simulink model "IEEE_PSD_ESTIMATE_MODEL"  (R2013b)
settings: Solver=ode45  StartTime=0.0  StopTime=SimulationDuration  RelTol=1e-3
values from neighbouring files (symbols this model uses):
  Amplitude = TypicalTransmitAmplitude * 0.95    (= 1.14)    [IEEE_PSD_ESTIMATE.m]
  Coefficients = [1 1 1 1 1 1] / 6    [IEEE_PSD_ESTIMATE.m]
  CouplingFilterFrequency = 8e6    (= 8000000)    [IEEE_PSD_ESTIMATE.m]
  DataRate = 10e6    (= 10000000)    [IEEE_PSD_ESTIMATE.m]
  Oversampling = 8    [IEEE_PSD_ESTIMATE.m]
  SymbolRate = DataRate * 3 / 4    (= 7500000)    [IEEE_PSD_ESTIMATE.m]
  Termination = 100    [IEEE_PSD_ESTIMATE.m]
  TransmitFilterFrequency = 12e6    (= 12000000)    [IEEE_PSD_ESTIMATE.m]
libraries: dspsigops x1, commrandsrc2 x1

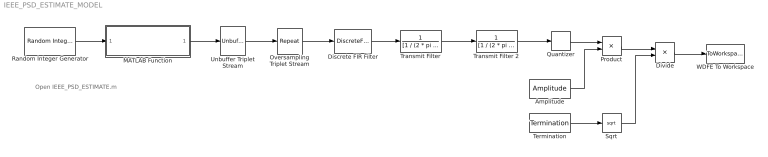
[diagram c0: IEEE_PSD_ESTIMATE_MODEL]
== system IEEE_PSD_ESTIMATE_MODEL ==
  note: Open IEEE_PSD_ESTIMATE.m
  Amplitude : Constant  Value=Amplitude
  Discrete FIR Filter : DiscreteFir  Coefficients=Coefficients
  Divide : Product  Inputs=*/
  MATLAB Function : MATLAB Function  TreatAsAtomicUnit=on
  Oversampling Triplet Stream : dspsigops/Repeat  N=16  RateOptions=Allow multirate processing  ic=0  mode=Unused parameter value
  Product : Product
  Quantizer : Quantizer  QuantizationInterval=1e-9  SampleTime=1 / (Oversampling * SymbolRate)
  Random Integer Generator : commrandsrc2/Random Integer Generator  mul=16  seed=37  Ts=4 / DataRate  frameBased=off  sampPerFrame=1  orient=off  outDataType=double
  Sqrt : Sqrt
  Termination : Constant  Value=Termination
  Transmit Filter : TransferFcn  Numerator=1  Denominator=[1 / (2 * pi * TransmitFilterFrequency) 1]
  Transmit Filter 2 : TransferFcn  Numerator=1  Denominator=[1 / (2 * pi * CouplingFilterFrequency) 1]
  Unbuffer Triplet Stream : Unbuffer  SampleBasedProcessing=Same as frame based
  WDFE To Workspace : ToWorkspace  VariableName=TX  SampleTime=-1
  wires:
  MATLAB Function/1(Triplet) -> Unbuffer Triplet Stream/1
  Unbuffer Triplet Stream/1 -> Oversampling Triplet Stream/1
  Random Integer Generator/1 -> MATLAB Function/1(Nibble)
  Oversampling Triplet Stream/1 -> Discrete FIR Filter/1
  Discrete FIR Filter/1 -> Transmit Filter/1
  Product/1 -> Divide/1
  Divide/1 -> WDFE To Workspace/1
  Amplitude/1 -> Product/2
  Termination/1 -> Sqrt/1
  Sqrt/1 -> Divide/2
  Transmit Filter/1 -> Transmit Filter 2/1
  Quantizer/1 -> Product/1
  Transmit Filter 2/1 -> Quantizer/1
